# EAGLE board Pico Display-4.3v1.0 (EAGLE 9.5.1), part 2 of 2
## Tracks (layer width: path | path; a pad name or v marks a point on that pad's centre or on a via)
+1V1  (via drill 0.35)
  Top 0.203: U1.50 37.86,33.68 37.86,32.15 39.06,30.94 v39.06,30.61 39.05,30.59 C13.1 | C16.1 33.43,44.09 34.8,44.09 37.06,41.83 37.06,41.3 37.06,41.05 U1.23
  Top 0.254: 37.06,41.3 37.06,40.3 36.59,39.84 36.41,39.84 35.13,38.56 35.13,35.29 35.86,34.56 U1.45 35.86,30.91 v35.52,30.58 35.28,30.34 C14.1
  Bottom 0.5: v39.06,30.61 38.56,30.11 36.25,30.11 35.78,30.58 v35.52,30.58
+3V3  (via drill 0.35, 0.5)  (11 unrouted)
  Top 0.2: U4.8 66.8,57.4 | 69.74,57.4 R53.1 | 28.95,41.17 v29.02,41.17 | v30.91,37.97 31.31,38.37 U1.33 | U3.P$36 64.49,33.41 64.49,33.03 | R46.2 83.7,11.81 R16.2 | U1.44 U1.43 | v64.57,29.55 64.6,29.52 66.96,29.52 C48.1 | R35.2 113.19,25.81 v112.27,25.81
  Top 0.203: U1.10 43.31,38.37 43.55,38.14 v43.69,38.14 v43.69,38.15 44.54,38.15 C10.1 | U1.49 U1.48 37.08,33.91 37.08,31.71 37.49,31.3 | 37.34,29.93 C11.1 37.54,29.73 v37.54,31.27 | C39.1 56.33,37.18 U3.P$12 | C8.1 34.24,44.65 34.77,44.65 37.46,41.97 U1.22 | U1.44 35.3,33.94 | C3.1 43.29,32.95 41.47,34.77 U1.1 | U1.43 35.06,34.44 34.73,34.77 U1.42 | R22.2 44.35,49.9 R21.2 | 64.49,33.03 64.49,31.75 v64.56,31.68
  Top 0.254: U3.P$57 66.59,41.58 68.48,43.47 | 50.24,8.94 C7.1 | 52.8,19.74 53.09,19.46 | R116.2 46.28,54.79 C24.2
  Top 0.3: C18.2 111.25,52.81 111.25,54.38 | 111.25,54.38 111.25,54.76 v110.24,54.76 | 98.73,60.78 101.67,57.83 R118.2 101.78,54.76 v104.14,54.76 | C40.1 68.48,43.78 68.48,43.47 | U13.P$5 111.51,54.64 111.25,54.38 | J10.5 20.91,41.07 | C8.1 34.24,45.16 34.77,45.16 v35.07,45.46 | v45.47,49.94 44.39,49.94 R22.2 | R16.2 84.26,11.76 85.34,12.85 85.34,14.12 84.33,15.14 76,15.14 74.83,16.31 74.83,19.43 74.31,19.95 C37.2
  Top 0.5: C12.1 v33.85,30.89 33.85,32.08 35.26,33.49 35.26,34.16 | J1.3 15.64,63.54 17.27,65.18 18.29,65.18 | 18.29,65.18 18.8,65.18 20.57,63.4 20.57,61.37 21.34,60.6 24.38,60.6 25.53,59.45 C36.1 C47.1 25.53,56.46 26.13,55.86 27.89,55.86 29.1,54.66 C5.1 | R3.2 49.43,55.97 R26.2 49.47,55.49 48.2,54.22 | v44.73,54.15 44.59,54.01 33.97,54.01 v33.76,54.23 31.71,54.23 31.26,54.68 C57.2 29.86,54.67 C5.1 | 31.35,56.96 R74.2 31.35,58.93 32.01,59.59 J2.3 | v71.12,58.06 70.46,57.4 69.74,57.4 66.8,57.4 66.7,57.3 64.77,57.3 63.45,58.62 55.42,58.62 54.31,57.51 R9.2 R19.2 54.31,55.49 53.46,54.64 53.46,54.63 52.3,53.47 50.05,53.47 49.11,54.42 C58.2 48.01,54.43 C24.2 46.6,54.4 44.97,54.4 v44.73,54.15 | 20.91,41.07 22.19,42.35 U10.8 23.38,43.79 C92.1 | C92.1 R1.2 25.18,45.62 13.46,45.62 12.19,44.35 U10.3 12.19,38.54 C90.2 11.39,36.15 C91.1 11.4,36.04 11.4,33.43 | 9.81,27.58 J5.3 15.75,27.62 C26.2 16.17,27.56 14.93,28.8 14.28,28.8 11.4,31.68 11.4,33.43 | R30.2 C38.1 52.46,34.66 C39.1 55.2,33.27 55.2,28.72 56.1,27.82 R36.2 56.12,25.75 56.49,25.38 R7.2 57.37,25.36 58.05,24.68 v58.05,23.8 | 98.73,60.78 98.73,64.24 97.79,65.18 94.49,65.18 93.4,64.08 J7.14 93.4,58.65 v93.47,58.57 v93.48,58.58 | U2.8 39.55,23.85 39.31,24.09 C15.1 C9.1 | C9.1 | v44.45,31.3 44.15,31.6 C3.1 | R27.2 50.24,8.94 | C7.1 50.64,8.88 53.09,11.33 53.09,19.46 | v39.22,26.64 39.31,26.55 C9.1 | C92.1 25.53,43.64 27.14,42.03 27.12,42 C27.1 27.3,41.17 v29.02,41.17 | C5.1 31.35,54.66 R73.2 31.35,55.86 | v69.44,54.57 69.72,54.29 69.72,45.89 68.6,44.77 C40.1 | 18.29,65.18 v18.29,65.68 | 11.4,33.43 11.14,33.17 v10.41,33.17
  Top 0.5: v44.73,54.15 44.8,54.22 | 49.43,57.72 48.51,58.64 48.51,61.94 J6.3 | v110.49,35.97 R85.2
  Top 0.8: C37.2 C41.2 C44.1 R57.1 R56.1 66.47,19.95 | 66.47,19.95 R59.1 66.42,19.95 | R60.1 62.53,19.77 | R60.1 R58.1 | SD2.4 65.95,16.97 65.2,17.72 65.2,19.95 | 67.1,29.45 C48.1 C49.1 67.07,27.15 66.45,26.54 66.45,26.31 66.47,26.29 R17.2 65.68,26.41 64.82,25.55 64.82,23.52 | C26.2 26.42,27.56 | 26.42,27.56 29.18,27.56 31.23,29.6 C12.1 | R74.2 R73.2 | 52.8,19.74 v58,19.74 36.8,19.74 34.04,22.5 28.45,22.5 26.42,24.54 26.42,27.56 | 59.09,23.75 58.15,23.75 | 64.82,23.52 74.16,23.52 R79.1 76.68,23.64 Q8.2 77.55,23.28 80.68,23.28 R87.1 82.4,24.13 84.07,25.81 87.12,25.81 87.78,25.15 R81.1 C88.1 C35.1 C34.1 93.71,24.57 C33.2 97.9,24.45 L1.2 98.15,22.72 v98.12,22.7 | 64.82,23.52 59.32,23.52 | 61.29,19.96 R58.1 | 61.1,19.74 R58.1 | R60.1 65.2,19.95 | 65.2,19.95 66.47,19.95 | R58.1 61.13,19.77 v58.91,19.77
  Top 1: 59.32,23.52 59.09,23.75
  Bottom 0.2: v30.91,37.97 28.98,39.89 28.98,41.13 v29.02,41.17 | v110.49,35.97 109.97,35.44
  Bottom 0.203: v37.54,31.27 37.49,31.21 35.26,31.21 | v64.56,31.68 64.53,31.65 64.53,29.59 v64.57,29.55
  Bottom 0.254: 109.09,25.76 109.13,25.81 v112.27,25.81
  Bottom 0.3: 45.47,49.68 v45.47,49.94 44.86,49.33 44.86,39.32 v43.69,38.14 | v104.14,54.76 v110.24,54.76
  Bottom 0.5: v93.47,58.57 92.46,59.59 72.64,59.59 v71.12,58.06 69.43,56.37 69.43,54.58 v69.44,54.57 | v33.76,54.23 34.02,53.97 34.02,46.46 35.02,45.46 v35.07,45.46 29.99,45.46 28.68,44.14 28.68,41.52 v29.02,41.17 | v44.73,54.15 44.73,51.18 45.47,50.45 v45.47,49.94 | v44.45,31.3 44.35,31.39 37.67,31.39 v37.54,31.27 37.41,31.39 34.36,31.39 v33.85,30.89 33.85,30.05 36.32,27.58 38.28,27.58 v39.22,26.64 | v10.41,33.17 9.65,32.41 PAD1.P$1 | v110.49,35.97 109.09,34.57 109.09,25.76 109.09,24.5 105.3,20.71 100.12,20.71 v98.12,22.7 | v18.29,65.68 PAD19.P$1
  Bottom 0.8: P13.P$1 57.89,23.64 v58.05,23.8
  other vias: 58.92,18.72 58.01,18.72 58.92,23.77 58.97,22.64 58.04,22.66
  pour Top: 57.71,24.09 57.71,22.56 57.9,22.37 59.16,22.37 59.31,22.51 59.31,24.14 59.03,24.42 58.04,24.42
  pour Bottom (no thermals): 57.46,23.84 57.46,18.77 57.87,18.37 59.12,18.37 59.49,18.74 59.49,23.96 59.03,24.42 58.04,24.42
  pour Top: 57.45,19.96 57.45,18.79 57.88,18.35 58.89,18.35 59.25,18.71 59.25,20.01 59.1,20.16 57.65,20.16
  pour Top: 24.64,27.84 28.19,27.84 28.45,27.58 26.67,25.81 26.16,25.81 24.64,27.33
  pour Top (no thermals): 16.51,27.33 12.95,27.33 12.7,27.58 14.05,28.93 15.41,28.93 16.51,27.84
  pour Top: 51.93,19.68 54.33,19.68 53.13,18.48
+5V  (via drill 0.35)  (7 unrouted)
  Top 0.5: D8.A 109.63,20.19
  Top 0.55: 113.82,18.96 114.63,18.96 115.82,17.77 115.82,15.35 114.65,14.17 113.56,14.17
  Top 0.6: 113.51,18.97 112.24,18.97 112.14,19.08 | 113.56,14.12 v112.27,14.12
  Top 0.8: 112.14,19.08 111.38,19.08
  Top 1: 111.38,19.08 110.19,20.26 D8.A 109.55,20.34 109.55,22.89
  Bottom 0.5: PAD28.P$1 112.27,15.65 v112.27,14.12
BAT+  (via drill 0.35)  (1 unrouted)
  Top 0.2: 97.79,38.29 v97.81,38.31
  Top 0.5: 108.78,30.89 109.22,30.89 | C19.2 101,37.39 Q19.3 97.79,38.29
  Top 0.8: 108.78,30.89 106.44,33.23 106.44,34.65 105.46,35.63 U26.3 105.28,36.52 C20.2 C19.2
  Top 1: D14.A 110.09,31.87 J16.P$1
  Bottom 0.2: PAD53.P$1 99.28,38.31
  Bottom 0.5: v97.81,38.31 99.28,38.31
BL-POWER  (via drill 0.35)
  Top 0.2: U3.P$25 60.06,32.22 v58.37,30.53 | R50.2 95.48,44.76 95.48,32.47 97.75,30.2 97.75,27.12 96.32,25.68 v95.48,25.68 | v93.66,17.12 v77.35,17.12
  Bottom 0.2: 95.48,25.61 v95.48,25.68 95.48,24.93 94.02,23.47 94.02,17.47 v93.66,17.12 | v58.37,30.53 58.37,30.13 57.2,28.96 53.12,28.96 51.19,27.02 51.19,17.5 51.75,16.94 58.66,16.94 62.08,20.36 71.94,20.36 75.11,17.19 77.28,17.19 v77.35,17.12
BL-PWM1
  Top 1: R101.2 R8.1 R4.1 R118.1
BOOT  (via drill 0.35)
  Top 0.2: R6.2 54.92,25.61 54.36,25.61 53.86,25.11 v53.86,24.83 | 107.66,2.09 116.8,11.22 116.8,22.51 118.44,24.15 118.44,25.8 116.44,27.79 116.44,48.2
  Top 0.203: v55.37,18.44 55.37,10.96 58.38,7.95 75.38,7.95 81.24,2.09 107.66,2.09
  Top 0.254: 116.44,48.2 115.33,49.32 SW2.2
  Bottom 0.203: v55.37,18.44 53.86,19.96 v53.86,24.83
BW16-RX
  Top 0.203: R109.2 23.5,53.1 13.01,53.1 9.69,56.42 9.69,57.9 U10.15
BW16-TX
  Top 0.203: U10.16 8.45,58.15 8.45,56.68 12.77,52.36 22.31,52.36 24.97,49.69 R108.2
CHG_LED
  Top 0.2: U26.1 107.46,37.17 D15.-
D+
  Top 0.203: R11.1 110.39,16.38 111.99,16.38 112.01,16.38 | J14.B6 112.78,17.32 112.42,17.32 112.01,16.92 112.01,16.38 | J14.A6 113.6,16.38 112.01,16.38
D-
  Top 0.203: R10.1 110.32,15.82 J14.B7 114.72,15.82 115.06,16.15 115.06,16.66 114.91,16.82 J14.A7
DVI5V
  Top 0.254: U3.P$9 54.54,38.38 C30.1
  Top 0.8: C30.1 R30.1 R31.1
DVI-CABLE-D  (via drill 0.35)
  Top 0.2: 58.06,31.27 56.87,31.27 56.75,31.39 v56.64,31.39 | R41.1 53.89,30.74 v54.05,30.58
  Top 0.203: U3.P$22 58.84,33.41 58.84,32.05 58.06,31.27
  Bottom 0.2: v54.05,30.58 54.86,31.39 v56.64,31.39
DVI-CABLE-DET
  Top 0.2: R40.1
  Top 0.5: R41.2 R40.1
DVI-CEC  (via drill 0.35)
  Top 0.2: 22.1,33.17 28.9,39.97 U1.29
  Top 0.203: v60.69,30.53 62.06,31.9 U3.P$30 | v52.03,17.73 40.22,17.73 v40.19,17.77 | 22.1,33.17 19.56,33.17 v18.8,33.93
  Bottom 0.203: v52.03,17.73 52.03,27.32 53.31,28.6 58.77,28.6 v60.69,30.53 | v18.8,33.93 18.8,31.14 24.89,25.04 32.91,25.04 v40.19,17.77
DVI-CLKN
  Top 0.2: U1.11 U3.P$8
DVI-CLKP
  Top 0.2: U3.P$7 U1.12
DVI-D0N  (via drill 0.35)
  Top 0.2: U1.13 43.59,39.57 44.4,40.39 44.4,41.02 43.97,41.45 42.92,41.45 v42.67,41.7 | v42.46,46.88 42.54,46.88 42.78,46.64 52.78,46.64 55.12,44.3 55.12,43.28 56.82,41.58 U3.P$1
  Bottom 0.2: v42.67,41.7 42.42,41.45 41.99,41.45 41.63,41.81 41.63,42.29 43.94,44.6 43.94,46.1 43.41,46.63 42.72,46.63 v42.46,46.88
DVI-D0P  (via drill 0.35)
  Top 0.2: U3.P$2 56.52,41.18 54.77,42.93 54.77,44.11 52.63,46.25 42.82,46.25 42.82,46.23 v42.57,45.98 | v42.67,40.79 42.67,40.89 42.82,41.05 43.69,41.05 43.97,40.77 43.97,40.49 43.43,39.95 41.11,39.95 U1.14
  Bottom 0.2: v42.57,45.98 42.57,46.03 42.77,46.23 43.23,46.23 43.51,45.95 43.51,44.68 41.28,42.45 41.28,41.58 41.81,41.05 42.42,41.05 v42.67,40.79
DVI-D1N  (via drill 0.35)
  Top 0.2: U3.P$3 56.09,40.78 53.78,43.09 47.35,43.09 v47.09,43.34 | U1.15 40.26,41.18 41.87,42.79 44.23,42.79 44.96,42.06 44.96,41.78 46.23,40.51 46.84,40.51 v47.17,40.18
  Bottom 0.2: v47.17,40.18 46.83,40.51 46.23,40.51 45.7,41.05 45.7,42.7 46.1,43.1 46.85,43.1 v47.09,43.34
DVI-D1P  (via drill 0.35)
  Top 0.2: U3.P$4 55.98,40.38 53.67,42.69 47.37,42.69 v47.09,42.41 | U1.16 39.86,41.28 41.76,43.18 44.6,43.18 45.44,42.34 45.44,41.82 46.37,40.89 46.91,40.89 v47.13,41.11
  Bottom 0.2: v47.13,41.11 46.89,40.87 46.41,40.87 46.05,41.23 46.05,42.44 46.3,42.7 46.85,42.7 47.09,42.45 v47.09,42.41
DVI-D2N  (via drill 0.35)
  Top 0.2: U1.17 39.5,40.86 39.5,41.62 42.48,44.59 51.86,44.59 v52.18,44.27 | U3.P$5 53.06,39.98 52.55,40.49 52.55,40.79 52.8,41.05 52.97,41.05 53.32,40.69 v53.32,40.66
  Bottom 0.2: v52.18,44.27 52.44,44.52 52.67,44.52 52.95,44.24 52.95,43.5 51.9,42.45 51.9,41.71 52.57,41.04 52.94,41.04 v53.32,40.66
DVI-D2P  (via drill 0.35)
  Top 0.2: U1.18 39.06,41.75 42.28,44.97 51.98,44.97 v52.19,45.18 | U3.P$6 52.95,39.58 52.15,40.39 52.15,40.99 52.56,41.4 53.14,41.4 v53.35,41.61
  Bottom 0.2: v52.19,45.18 52.46,44.91 52.87,44.91 53.46,44.31 53.46,43.37 52.36,42.27 52.36,41.83 52.77,41.43 53.17,41.43 v53.35,41.61
DVI-HPD  (via drill 0.35)
  Top 0.203: U1.35 32.19,37.57 30.37,35.76 28.34,35.76 23.85,31.27 v21.34,31.27 | v78.23,7.01 78.23,10.53 Q2.3 80.52,10.56 R43.1 C51.1
  Bottom 0.2: v21.34,31.27 26.67,25.94 33.53,25.94
  Bottom 0.203: 33.53,25.94 52.45,7.01 v78.23,7.01
DVI-HPD0  (via drill 0.35)
  Top 0.2: v82.08,14.2 82.19,14.09 R44.2 | U3.P$63 63.26,43.36 64.15,44.25 65.04,44.25 67.31,46.52 v67.31,47.84
  Top 0.254: R44.2 83.67,13.21 R16.1 | v86.48,14.04 86.52,14 v96.46,14
  Bottom 0.254: v67.31,47.84 67.4,47.74 78.47,47.74 78.96,48.23 96.08,48.23 102.36,41.95 102.36,36.74 99.36,33.74 99.36,25.55 95.9,22.09 95.9,14.56 v96.46,14 | v82.08,14.2 86.32,14.2 v86.48,14.04
EN-TP  (via drill 0.35)
  Top 0.2: U3.P$60 64.46,42.95 64.62,43.1 | 29.5,48.7 28.92,48.12 27.09,48.12 R18.2 | 65.99,43.1 66.66,43.1 67.21,43.66 67.21,44.82 68.61,46.22 | 29.5,50.89 30.2,51.59 32.84,51.59 33.68,52.43 42.46,52.43 43.17,51.72 53.6,51.72
  Top 0.203: 64.62,43.1 65.99,43.1 | 29.5,48.7 29.5,50.89 | v63.47,53.02 54.9,53.02 53.6,51.72 | v68.37,52.84 68.61,52.6 68.61,46.22
  Bottom 0.203: v63.47,53.02 68.19,53.02 v68.37,52.84
EN_RESET  (via drill 0.35)
  Top 0.2: U3.P$61 64.06,43.13 64.4,43.47 | v67.92,48.61 67.96,48.57 67.96,46.23 66.79,45.05 66.79,43.75 66.51,43.47 | R88.2 75.18,35.93 78.08,38.82 78.08,48.29 v78.22,48.43
  Top 0.203: 66.51,43.47 64.4,43.47
  Bottom 0.2: v78.22,48.43 68.1,48.43 v67.92,48.61
FLASH-WP  (via drill 0.35)
  Top 0.2: U3.P$58 66.68,42.53 67.56,43.42 67.56,44.53 69.19,46.16
  Top 0.203: v68.35,55.02 68.35,53.97 69.19,53.13 69.19,46.16 | R20.2 R19.1 56.56,54.87 56.61,54.86 U4.3 58.78,55.11 61.94,55.11 v62.08,54.97
  Bottom 0.203: v68.35,55.02 68.3,55.07 62.17,55.07 v62.08,54.97
GND  (via drill 0.35)  (492 unrouted)
  Top 0.203: C28.2 53.66,49.49 v53.59,49.43 | X1.2 39.91,48.99 40.69,48.2 40.69,44.66 38.66,42.62 U1.19 38.66,38.37 U1.EPAD | C16.2 C8.2 34.59,46.43 v35.13,46.96 | v38.1,44.09 38.02,44.17 C1.2 38.02,46.75 X1.4 39.69,48.49 X1.2 | X1.2 39.97,49.28 v41.45,49.28 42.43,49.28 R23.2 43.12,49.85 43.82,49.15 45.65,49.15 C6.2 47.29,49.2 48.28,49.2 48.98,49.9 C25.2 C21.2 51.85,49.9 v52.32,49.43 | C47.2 C36.2 27.06,59.71 v26.67,60.1 | C57.1 C5.2 | R15.1 27.33,53.57 v28.06,54.3 | C4.2 28.16,45.62 v28.96,45.62 | C92.2 28.53,42.32 v30.59,42.32 | v26.8,39.85 26.74,39.85 C27.2 23.36,38.76 v22.1,38.76
  other vias: 60.35,45.8 63.47,47.9 62.55,50.81 53.74,52.98 55.44,50.87 54.1,48.16 55.98,46.79 58.17,45.62 60.68,51.13 58.93,37.85 58.93,40.74 38.1,65.68 24.89,23.01 31.5,20.98 9.65,50.95 14.48,17.93 35.81,51.21 9.55,48.46 36.93,43.41 59.44,46.71 35.1,48.69 21.89,50.04 45.52,18.8 35.16,61.57 56.96,43.15 14.27,18.9 40.18,50.55 41.25,47.27 38.05,51.41 52.02,12.8 69.25,42.86 70.1,41.07 71.88,40.31 73.66,39.55 75.07,38.62 39.88,43.82 70.61,16.66 72.14,16.66 73.66,16.66 36.83,16.66 36.58,12.85 36.32,8.53 52.32,5.74 50.8,3.71 42.16,14.38 50.29,5.99 11.94,19.46 9.4,39.27 9.4,34.44 18.8,63.4 35.73,65.36 40.49,62.52 38.74,62.54 9.65,53.75 50.29,59.59 57.86,51.28 56.9,54 95.76,63.91 100.84,60.86 102.26,60.76 100.84,63.14 102.62,63.14 103.63,60.86 113.18,62.53 111.66,66.34 113.44,59.23 103.28,56.69 109.37,50.09 101.5,46.28 97.98,47.68 105.31,42.72 97.69,43.23 105.31,38.4 106.58,38.4 107.53,35.02 106.58,37.39 97.69,35.86 97.55,34.39 113.18,24.69 111.91,21.39 113.18,21.89 111.91,22.91 113.18,23.42 20.78,25.4 18.64,25.4 111.91,24.18 112.93,10.97 110.77,11.32 111.19,13.17 103.3,13.9 99.9,14.6 97.25,14.7 107.95,11.28 85.46,10.21 108.67,7.46 111.03,9.25 105.82,17.32 105.36,13.97 84.86,24.28 92.1,21.89 97.19,21.88 84.99,19.61 87.27,18.59 91.71,15 100.48,10.72 99.21,10.72 83.46,8.69 69.93,28.19 75.19,28.61 73.76,27.18 67.14,31.87 53.37,25.95 55.99,32.12 55.02,37.13 44.7,30.1 45.87,36.88 39.01,22.91 32.41,27.74 31.14,27.74 37.74,26.72 57.66,11.84 50.55,22.25 75.91,13.95 80.52,18.44 44.2,22.76 31.75,31.14 37.36,36.86 38.63,36.86 36.09,38.25 36.09,36.89 58.93,34.95 22.35,56.54 16.76,55.27 11.94,56.29 18.03,50.44 9.65,45.87 49.78,64.67 102.36,59.08 104.67,35.01 113.18,36.37 113.18,35.36 113.18,37.64 113.18,30.53 113.18,29.26 113.18,27.74 75.97,66.34 62.84,54.34 67.65,52.04 89.41,63.65 74.17,65.18 71.37,64.67 69.09,64.67 30.48,59.59 16.26,44.6 100.84,28.85 89.05,3.61 107.09,3.61 110.39,6.15 75.59,3.1 101.5,29.51 37.36,35.53 39.9,35.53 60.33,37.85 60.32,40.74 60.33,34.95 63.12,37.85 63.1,40.74 63.12,34.95 64.52,37.85 64.49,40.74 64.52,34.95 63.1,39.29 64.49,39.29 63.1,36.4 64.49,36.4 60.32,36.4 60.32,39.29 58.93,39.29 58.93,36.4 38.63,35.53 36.09,35.53 61.71,40.74 61.71,39.29 61.72,37.85 61.71,36.4 61.72,34.95 39.9,36.86 39.9,38.19 39.9,39.52 38.63,38.19 37.36,38.19 38.61,39.52 37.36,39.52 63.68,26.25 67.6,36.61 56.53,18.62 57.33,17.75 50.55,18.69 49.28,22.5 54.1,17.68 53.34,7.77 54.36,7.77 53.59,9.55 57.66,13.36 54.1,12.6 85.44,15.09 36.07,3.45 55.63,3.45 66.04,3.45 85.34,4.47 29.74,23.49 31.04,23.44 20.95,44.42 17.65,39.09 20.45,31.72 16.64,31.72 27.18,30.89 25.98,30.61 75.95,11.33 92.86,10.48 100.32,27.36 94.47,35.36 93.01,32.35 84.46,32.5 80.75,32.38 113.28,49.94 108.71,67.72 89.92,68.48 97.79,68.73 82.55,68.73 108.86,61.01 94.23,56.79 94.23,55.27 96.77,56.79 98.55,55.78 97.03,55.52 96.27,53.24 79.25,52.73 82.13,42.75 80.81,40.62 84.36,40.62 87.67,40.62 91.44,40.76 80.84,36.07 84.36,36.08 88.02,36.07 84.7,46.47 98.63,53.42 86.24,43.1 45.97,39.85 54.36,40.63 54.13,43.65 45.8,43.69 52.12,48.01 44.12,43.82 55.69,44.91 35.18,32.26 45.59,24.13 47.97,15.38 63.73,24.7 55.88,64.16 60.45,64.16 93.11,46.82 35.37,39.77 76.53,21.03 83.49,18.97 81.6,19.81 92.59,17.81 46.21,33.21 36.42,54.82 40.79,54.85 46.01,58.63 56.22,22.29 88.87,15.01 52.96,22.67 62.48,24.74 51.4,34.32 56.06,30.43 65.21,28.41 69.03,31.87 67.14,33.52 92.61,8.2 99.79,8.34 105.42,10.62 105.36,8.24 70.79,36.68 77.96,34.58 57.25,30.6 91.52,36.2 62.4,26.33 76.17,35.88 98.67,32.29 89.67,43.09 93,42.99 88.03,32.39 68.02,41.95 70.16,45.17 71.87,46.36 71.87,54.38 67.65,49.87 71.87,49.23 55.64,35.51 55.64,34.11 62.53,31.07 64.46,27.39 62.71,27.78 71.63,42.62 73.1,41.57 74.46,40.41 75.97,39.54 78.24,37.87 62.73,29.28 61.61,46.85 51.81,39.83 56.21,43.96 57.46,32.5 32.46,40.71 30.64,40.82 32.6,32.17 28.72,32.29 67.7,35.11 70.89,33.64 69.11,33.57 70.86,35.14 69.17,36.68 80.77,34 80.74,38.34 84.38,38.34 87.74,38.52 91.52,38.55 84.38,34.28 87.95,34.14 69.21,35.21 83.07,22.98 84.72,22.95 75.83,27.74 72.68,24.52 71.09,28.16 78.83,35.04 69.83,29.28 78.91,22.14
  pour Bottom (rank 2, no thermals): 7.87,69.62 113.79,69.62 113.79,1.93 7.87,1.93
  pour Top (rank 2, no thermals): -0.25,72.03 122.17,72.03 122.17,-0.61 0,-0.61 0,33.68 7.87,33.68 7.87,65.43 -0.25,65.43
GP0/UART0_TX  (via drill 0.35)
  Top 0.2: J7.1 56.24,60.95 56.14,60.85
  Top 0.203: U1.2 41.58,35.17 45.48,31.26 46.61,31.26 48.51,29.36 48.51,28.81 v49.24,28.08 | v51.82,54.25 52.53,54.97 R70.1 53.35,56.25 53.35,58.07 56.14,60.85
  Bottom 0.2: v51.82,54.25 53.99,56.42 PAD44.P$1
  Bottom 0.203: v49.24,28.08 49.9,28.74 49.9,50.68 51.56,52.34 51.56,54 v51.82,54.25
GP1/UART0_RX  (via drill 0.35)
  Top 0.2: 62.92,62.2 J7.2
  Top 0.203: U1.3 41.73,35.57 45.59,31.71 46.77,31.71 49.2,29.29 v49.2,29.03 | v50.8,54.25 51.13,54.59 R83.1 50.67,55.4 50.29,55.78 50.29,58.45 55.09,63.25 61.87,63.25 62.92,62.2
  Bottom 0.2: v50.8,54.25 50.8,54.95 PAD43.P$1
  Bottom 0.203: v50.8,54.25 50.8,52.73 49.51,51.44 49.51,29.34 v49.2,29.03
GP2/I2C1_SDA  (via drill 0.35)  (1 unrouted)
  Top 0.2: v65.3,58.65 v65.29,58.65 65.46,58.81 J7.3 65.46,64.34 | U1.4 41.9,35.97 45.77,32.1 47.02,32.1 50.02,29.11 50.41,29.11 v50.61,28.91 | 65.46,64.34 65.53,64.41 | 65.46,64.34 65.46,64.49 v65.28,64.67 | 46.37,62.09 J6.2 | R121.1 v38.49,55.84 v38.5,55.83 39.13,55.83 Q5.3 | J6.2 46.5,65.66 v46.37,65.79 | J6.2 46.5,59.83 47.91,58.43 R3.1
  Top 0.203: R3.1 48.16,57.65
  Bottom 0.2: v65.28,64.67 62.99,66.95 47.53,66.95 | 47.53,66.95 47.52,66.95 | v38.5,55.83 37.06,55.83 36.47,56.42 36.47,61.95 39.83,65.31 45.88,65.31 v46.37,65.79 | v46.37,65.79 | v46.37,65.79 47.53,66.95 | v50.61,28.91 50.63,28.93 50.34,29.23 50.34,50.62 52.19,52.48 52.19,53.57 59.39,60.76 63.18,60.76 v65.3,58.65
GP2/I2C1_SDA-5V  (via drill 0.35)
  Top 0.2: U3.P$71 60.06,44.2 63.14,47.27 63.74,47.27 64.11,47.64 64.11,50.24 62.36,51.99 55.45,51.99 54.38,50.93 41.58,50.93 v41.54,50.96
  Top 0.254: R45.1 41.92,57.42 41.92,58.14 v41.55,58.51 | R121.2 Q5.2 38.73,58.58 v38.78,58.63
  Bottom 0.2: v41.55,58.51 41.51,58.47 41.51,51 v41.54,50.96
  Bottom 0.254: v41.55,58.51 41.36,58.7 38.85,58.7 v38.78,58.63
GP3/I2C1_SCL  (via drill 0.35)  (1 unrouted)
  Top 0.2: v67.92,64.59 67.92,61.37 | 67.92,61.37 67.92,61.03 J7.4 | 47.14,58.46 44.75,60.85 44.75,61.71 J6.1 44.5,65.46 | U1.5 42.01,36.37 45.86,32.53 47.22,32.53 50.12,29.62 50.8,29.62 v51.55,28.88 | v67.56,58.57 68.07,59.08 68.07,61.21 67.92,61.37 | R122.1 34.69,55.84 35.07,55.45 Q9.3
  Top 0.203: R26.1 47.14,56.74 47.14,58.46 | 44.5,65.46 44.5,65.74 v44.7,65.94
  Bottom 0.2: 51.68,28.75 v51.55,28.88 50.75,29.68 50.75,50.53 52.55,52.33 52.55,53.39 59.5,60.34 62.55,60.34 64.87,58.02 67.03,58.02 67.56,58.55 v67.56,58.57 | v33.98,55.83 35.31,55.83 35.95,56.46 35.95,62.09 39.79,65.94 v44.7,65.94
  Bottom 0.203: v67.92,64.59 64.68,67.83 46.6,67.83 v44.7,65.94 43.73,65.94 PAD13.P$1
  Bottom 0.254: v44.7,65.94 44.81,65.94
GP3/I2C1_SCL-5V  (via drill 0.35)
  Top 0.2: U3.P$70 60.45,42.54 60.45,44.05 63.19,46.79 63.87,46.79 64.53,47.45 64.53,50.94 62.99,52.48 55.12,52.48 53.98,51.34 42.59,51.34 42.3,51.63 v42.25,51.57
  Top 0.254: v42.85,60.68 35.44,60.68 32.83,58.07 R122.2 Q9.2 | R47.1 43.41,58.23 v43.12,58.52
  Bottom 0.2: v42.25,51.57 42.25,58.01 42.76,58.52 v43.12,58.52 43.12,60.48 42.92,60.68 v42.85,60.68
GP4/UART1_TX  (via drill 0.35)
  Top 0.203: U1.6 42.4,36.77 45.23,33.95 45.66,33.95 v45.81,34.1 | v28.2,50.92 27.06,50.92 R109.1 27.17,51.19
  Bottom 0.203: v28.2,50.92 25.4,48.11 25.4,39.78 32.2,32.98 44.26,32.98 45.38,34.1 v45.81,34.1
GP5/UART1_RX  (via drill 0.35)
  Top 0.203: U1.7 42.62,37.17 44.53,35.26 45.11,35.26 v45.36,35 | v28.17,49.55 27.2,49.55 R108.1
  Bottom 0.203: v45.36,35 45.36,34.75 44.04,33.43 43.59,33.43 43.57,33.41 32.27,33.41 26.16,39.52 26.16,47.55 v28.17,49.55
GP6/SPI_CLK/SD_CLK  (via drill 0.35)
  Top 0.2: 70.54,64.41 J7.5
  Top 0.203: U1.8 42.72,37.57 44.45,35.84 47.37,35.84 v47.75,35.46 | SD2.5 64.8,15.29 v64.8,16.66 | 70.54,64.41 69.64,65.3 54.99,65.3 53.09,63.4 v51.82,63.4
  Bottom 0.2: 64.8,16.82 v64.8,16.66 64.72,16.66 PAD4.P$1
  Bottom 0.203: 64.86,16.72 v64.8,16.66 | 64.8,16.82 64.25,17.37 60.84,17.37 59.11,15.64 50.73,15.64 47.75,18.62 v47.75,35.46 47.75,36.34 48.67,37.25 48.67,50.55 47.5,51.71 47.5,54.51 51.82,58.83 v51.82,63.4
GP7/SPI_MOSI/SD_SDI  (via drill 0.35)
  Top 0.2: J7.6 73.08,64.74 72.9,64.92
  Top 0.203: U1.9 42.93,37.97 44.65,36.25 48.69,36.25 v48.72,36.21 | SD2.3 v67.05,16.56 67.05,17.51 66.44,18.12 R59.2 | v52.68,64.69 53.92,65.94 71.88,65.94 72.9,64.92
  Bottom 0.203: v67.05,16.56 67.05,17.17 66.33,17.89 62.48,17.89 | 62.48,17.89 60.75,17.89 58.97,16.11 50.88,16.11 48.51,18.48 48.51,36 v48.72,36.21 49.05,36.54 49.05,51.31 48.06,52.3 48.06,54.36 52.68,58.98 v52.68,64.69 | PAD3.P$1 62.48,17.89
GP16/SPI_MISO/SD_SDO  (via drill 0.35)  (1 unrouted)
  Top 0.2: U1.27 35.46,41.28 35.13,41.61 33.42,41.61 30.93,44.09 30.93,48.87 v31.5,49.43 | 75.55,65.24 75.55,61.02 J7.7
  Top 0.203: SD2.7 v62.65,16.66 62.65,18.37 R60.2 | 75.55,65.24 73.89,66.9 34.75,66.9 v34.04,66.19
  Bottom 0.2: v34.04,66.19 31.94,64.1 31.94,49.88 v31.5,49.43 27.81,45.75 27.81,39.4 33.02,34.19 42.93,34.19 44.86,36.12 46.08,36.12 47.37,34.82 47.37,18.29 50.52,15.14 61.12,15.14 v62.65,16.66
GP17/SD_CS/SPI_CS2  (via drill 0.35)
  Top 0.2: U1.28 35.06,41.09 34.93,41.22 33.24,41.22 30.58,43.88 30.58,49.78 v31.24,50.44 | 78.09,64.92 78.09,61.73 77.98,61.62 77.98,61.13 J7.8
  Top 0.203: SD2.2 68.2,15.28 v68.2,16.56 68.2,17.88 68.22,17.9 67.86,18.25 R56.2 | 78.09,64.92 78.09,65.66 76.36,67.38 34.33,67.38 33.52,66.57 v32.94,66.57
  Bottom 0.2: v32.94,66.57 31.24,64.87 v31.24,50.44 27.43,46.63 27.43,39.01 32.68,33.77 43.01,33.77 45.01,35.77 45.9,35.77 46.96,34.7 46.96,18.01 50.25,14.72 67.66,14.72 68.2,15.26 v68.2,16.56
  Bottom 0.203: v68.2,16.56 69.09,17.45 PAD2.P$1
GP19/BUZZER  (via drill 0.35)  (1 unrouted)
  Top 0.2: 28.71,39.26 28.69,39.26 22.25,32.82
  Top 0.203: v17.53,33.17 17.88,32.82 22.25,32.82 | R28.2 39.85,12.66 39.85,15.37 39.85,15.67 v39.37,16.15 | U1.30 29.01,39.57 28.98,39.53 28.72,39.28 28.71,39.26
  Bottom 0.203: v17.53,33.17 17.53,31.14 24.38,24.28 31.75,24.28 39.37,16.66 v39.37,16.15
GP20/I2C0_SDA  (via drill 0.35)
  Top 0.203: U1.31 29.32,39.17 23.34,33.2 23.07,32.92 v23.07,32.67 | J10.1 18.91,36.87 v20.57,35.2
  Bottom 0.2: v23.07,32.67 24.34,31.39 PAD52.P$1
  Bottom 0.203: v23.07,32.67 23.07,32.71 v20.57,35.2
GP21/I2C0_SCL  (via drill 0.35)
  Top 0.203: U1.32 29.83,38.77 v24.03,32.97 | J10.2 19.41,37.64 v20.07,36.98
  Bottom 0.2: PAD16.P$1 20.57,37.49 v20.07,36.98
  Bottom 0.203: v20.07,36.98 20.07,36.68 23.77,32.97 v24.03,32.97
GP22-PWM  (via drill 0.35)  (2 unrouted)
  Top 0.203: J5.1 14.83,23.62 v14.99,23.77 | U1.34 31.88,37.97 30.09,36.19 28.14,36.19 24.13,32.18 24.13,32.16 23.62,31.65 21.85,31.65 21.14,32.36 16.9,32.36 16.82,32.36 v15.49,33.68 | v81.03,67.01 81.03,61.62 80.77,61.37 80.77,61.01
  Bottom 0.203: v14.99,23.77 14.99,25.3 15.49,25.81 v15.49,33.68 15.49,66.19 18.03,68.73 78.49,68.73 80.21,67.01 v81.03,67.01
GP26*ADC0*I2C1_SDA  (via drill 0.35)
  Top 0.2: 83.32,63.24 83.32,61.03 J7.10 | R74.1 29.75,57.41 29.75,61.7 J2.2 29.97,61.99 29.97,63.78 v29.82,63.93 29.9,63.86 40.66,63.86 v40.95,64.14
  Top 0.203: U1.38 32.74,36.37 30.1,33.73 29.36,33.73 v29.21,33.58 | 83.32,63.24 83.31,63.24 v83.31,63.78
  Bottom 0.2: v29.82,63.93 29.82,62.99 PAD8.P$1
  Bottom 0.203: v29.82,63.93 27.71,63.93 23.77,59.99 23.77,37.34 27.53,33.58 v29.21,33.58 | v40.95,64.14 47.3,64.14 48.92,65.76 60.51,65.76 63.07,63.2 82.73,63.2 v83.31,63.78
GP27*ADC1*I2C1_SCL  (via drill 0.35)
  Top 0.2: 29.52,56.35 R73.1 28.01,57.86 28.01,61.62 | J2.1 28.19,62.14 v28.19,64.92 28.52,64.59 31.06,64.59 31.45,64.21 39.76,64.21 v40.1,64.54 | 86.11,63.35 86.11,61.28 J7.11
  Top 0.203: U1.39 32.9,35.97 29.86,32.93 27.67,32.93 v27.64,32.89 | 28.01,61.62 J2.1 | v28.19,64.92 28.25,64.86 | v86.11,63.91 86.11,63.35 86.11,62.89
  Bottom 0.2: v28.19,64.92 27.93,65.19 PAD9.P$1
  Bottom 0.203: v28.19,64.92 23.29,60.02 23.29,37.18 27.58,32.89 v27.64,32.89 | v40.1,64.54 40.35,64.8 47.21,64.8 48.6,66.19 60.96,66.19 63.5,63.65 81.28,63.65 82.04,64.41 85.6,64.41 v86.11,63.91
  Bottom 0.5: PAD9.P$1
GP28-ADC3  (via drill 0.35)  (3 unrouted)
  Top 0.203: J1.1 11.64,62.85 12.06,63.27 v12.06,64.54 12.06,66.07 13.79,67.79 86.79,67.79 88.14,66.45 88.14,61.72 | 34.18,35.56 33.09,35.56 27.39,29.87 15.31,29.87 v13.02,32.16
  Bottom 0.203: v13.02,32.16 13.08,32.21 13.08,61.75 12.06,62.76 v12.06,64.54
LVDS-POWER  (via drill 0.35)
  Top 0.2: v67.39,25.62 66.65,24.89 R17.1
  Top 0.203: U3.P$59 64.86,41.99 65.5,41.36 65.5,34.13 65.92,33.71 65.92,31.75 v65.95,31.71
  Top 0.3: v67.39,25.62 67.53,25.62 R80.2
  Bottom 0.2: v65.95,31.71 65.95,28.18 67.39,26.74 v67.39,25.62
LVDS-RESET  (via drill 0.35)  (2 unrouted)
  Top 0.3: J3.21 84.81,51.59 79.07,45.84 79.07,37.53 78.01,36.47 | C72.1 72.3,33.02 72.3,32.97
  Top 0.35: v77.96,36.49 76.02,34.55 C72.1 73.71,34.55 R88.1
  Bottom 0.2: v77.96,36.49 77.98,36.47 PAD39.P$1
LVDS_3V3  (via drill 0.5)  (1 unrouted)
  Top 0.2: 77.08,31.28 77.08,31.27 77.47,30.89
  Top 0.3: J3.3 J3.2
  Top 0.5: R96.2 73.87,31.41 | R89.2 74.12,33.17 v74.93,33.17
  Top 0.8: R87.2 80.62,25.66 Q8.3 79.59,25.31 77.08,27.82 77.08,31.27 | 73.87,31.41 R89.2 | 94.08,53.09 94.08,36.83 88.55,31.3 77.47,31.3 77.47,30.89 | R96.2 74.01,31.31 77.08,31.28
  Bottom 0.5: PAD21.P$1 v74.93,33.17
  pour Top: 75.95,31.39 78.42,31.39 77.18,30.16
LVDS_LEDA+  (via drill 0.5)  (1 unrouted)
  Top 0.3: J3.25 J3.24 J3.23
  Top 0.6: U5.5 104.74,45.53 v104.65,45.62 | 107.45,52.98 C53.2 C55.2 107.69,51.14 v107.69,50.08 107.69,48.29 D6.C | v104.9,52.98
  Top 0.8: 107.45,52.98 v104.9,52.98
  Top 1: J3.24 v83.31,51.46
  Bottom 0.6: v104.65,45.62 104.65,47.04 v107.69,50.08
  Bottom 0.8: v104.9,52.98 103.38,51.46 v83.31,51.46
LVDS_LEDK-  (via drill 0.5)  (1 unrouted)
  Top 0.2: 100.76,48.97 R99.2
  Top 0.3: J3.29 J3.28 81.53,52.86 J3.27
  Top 0.8: R98.1 102.28,47.46 100.76,48.97 | R99.2 R48.1
  Top 1: J3.28 81.31,49.97 v81.28,49.94 | R99.2 99.39,48.97 98.63,49.73 v98.63,50.06
  Bottom 1: v98.63,50.06 98.45,49.89 81.33,49.89 v81.28,49.94
N$1
  Top 0.203: X1.3 37.32,48.32 C2.2 R2.1
N$2
  Top 0.203: U1.21 37.86,43.4 36.44,44.82 R2.2
N$3
  Top 0.203: U1.20 38.26,43.23 39.55,44.52 C1.1 39.55,46.65 X1.1
N$5
  Top 0.203: J15.B5 106.64,60.26 R68.1
N$8  (via drill 0.35)
  Top 0.2: J3.20 85.31,51.46 79.67,45.82 79.67,34.37 v78.82,33.51
  Top 0.35: R55.1 71.96,31.39 v71.1,32.25
  Bottom 0.2: 78.89,33.58 v78.82,33.51 78.82,32.85 77.77,31.8 71.55,31.8 v71.1,32.25
N$9
  Top 0.2: R84.1 108.8,33.81 U26.5
N$10
  Top 0.8: U6.3 97.21,20.82 L1.1
N$14
  Top 0.2: U4.7 69.48,56.13 R53.2
N$15
  Top 0.2: D15.+ 110.5,38.69 R85.1
N$16
  Top 0.203: J15.A5 109.64,61 R69.2
N$23  (1 unrouted)
  Top 0.254: Q4.1 40.08,10.87 39.88,11.07 | R29.2 39.62,10.88 R28.1
N$27
  Top 0.2: R32.1 100.07,34.79 | Q19.1 99.99,36.39
  Top 0.5: R66.2 R32.1
  Top 0.8: Q19.1 100.19,36.37 R66.2
N$28
  Top 0.203: R12.1 110.32,18.32 J14.B5
N$29  (1 unrouted)
  Top 0.254: Q4.3 39.19,7.22 40.01,7.22 42.3,7.22 | 42.55,10.15 D2.A
  Top 0.5: D2.A 42.53,7.66 42.93,7.26 42.77,7.26 B1.2
N$30
  Top 0.254: R27.1 48.68,7.22 | 46.56,10.16 D2.C
  Top 0.5: R27.1 46.62,7.41 B1.1 46.55,10.15 46.56,10.16
N$31
  Top 0.2: U5.3 103.82,46.99
  Top 0.8: 103.82,46.99 103.82,48.91 R100.1 104.11,49.23 102.68,49.23 R98.2
N$32
  Top 0.203: R13.2 111.08,14.21 112.19,15.32 J14.A5
N$35
  Top 0.3: R35.1 D3.+
N$36
  Top 0.203: R57.2 69.34,18.38 69.34,15.32 SD2.1
N$43  (via drill 0.35)
  Top 0.3: R82.2 R81.2 C88.2 89.86,22.25 89.92,22.25 v89.83,22.16 | v90.32,19.69 90.34,19.69 U6.5
  Bottom 0.3: v89.83,22.16 90.32,21.66 v90.32,19.69
N$49
  Top 0.2: 104.14,50.74 R100.2
  Top 0.8: R101.1 104.14,50.75
  Top 1: 104.14,50.75 104.14,50.74 | R100.2 C73.1
N$50
  Top 0.3: C17.2 113.28,53.49 113.28,58.06 112.9,58.45 U13.P$8
N$51
  Top 0.2: U3.P$29 61.66,32.58 59.88,30.8 59.88,29.63 R38.1
  Top 0.203: U3.P$29 61.64,33.41 | 61.64,29.73 61.33,29.41 R39.2 R38.1
N$52
  Top 0.203: U3.P$23 59.26,33.41
N$57
  Top 0.203: R58.2 61.31,15.47 SD2.8
N$67
  Top 0.203: U3.P$74 58.84,42.55 58.84,43.7 56.42,46.13 55.12,46.13 53.85,47.4 52.51,48.73 50.81,48.73 C21.1 | 48.05,48.63 R21.1 C21.1 | C21.1 C25.1
N$70
  Top 0.5: U5.1 105.74,46.96 105.99,46.71
  Top 1: D6.A 111.91,47.52 L4.2 107.32,45.38 105.99,46.71
N$71
  Top 0.8: Q1.1 98.94,42.82 100.84,42.82 102.1,44.08 Q3.3
  Top 1: Q1.1 96.77,42.11 R49.2
N$73
  Top 0.2: Q3.1 98.39,46.07 R51.2 98.02,45.78 R50.1
N$76
  Top 0.203: R15.2 25.61,53.57 R5.1
N$101
  Top 0.203: U3.P$26 60.46,31.98 59.24,30.76 59.24,29.7 R37.1 57.19,29.35 57.21,29.37 C50.1 56.14,29.37 R36.1
N$102
  Top 0.2: C29.2 R24.1 60.9,49.43 59.51,49.43 X2.3
N$103
  Top 0.2: U3.P$75 58.46,43.29 56.13,45.62 55.04,45.62 53.31,47.35 45.28,47.35 R22.1
  Top 0.203: R23.1 R22.1
N$105
  Top 0.2: R78.1 103.79,42.19 U5.4
N$121
  Top 0.5: Q11.3 74.82,25.71 R79.2 76.2,25.64 Q8.1
N$122
  Top 0.5: Q11.1 71.11,26.37 R86.2 69.65,26.39 R80.1
QSPI_CS  (via drill 0.35)
  Top 0.203: U1.56 40.26,33.68 41.99,31.95 41.99,29.72 42.6,29.11 44.22,29.11 45.47,27.86 45.47,26.82 46.48,25.81 v49.68,25.81 | v49.78,23.77 49.78,23.85 U2.1 51.84,23.61 54.95,23.61 R6.1 R7.1
  Bottom 0.203: v49.68,25.81 49.68,23.88 v49.78,23.77
QSPI_D0
  Top 0.203: U2.5 43.24,27.41 41.52,27.41 40.83,28.1 40.83,31.24 39.06,33.02 U1.53
QSPI_D1
  Top 0.203: U2.2 46.04,25.12 44.96,26.2 44.96,27.84 44.2,28.6 42.42,28.6 41.59,29.43 41.59,31.54 39.86,33.28 U1.55
QSPI_D2  (via drill 0.35)
  Top 0.203: U1.54 39.46,33.17 41.23,31.4 41.23,28.87 v41.86,28.24 | U2.3 50.83,26.39 50.38,26.85 47.98,26.85 45.62,29.21 v45.52,29.21
  Bottom 0.203: v45.52,29.21 44.55,28.24 v41.86,28.24
QSPI_D3
  Top 0.203: U1.51 38.26,32.54 40.03,30.76 40.03,27.68 42.67,25.04 43.41,25.04 U2.7
QSPI_SCK
  Top 0.203: U1.52 38.66,32.79 40.43,31.01 40.43,27.89 41.93,26.39 U2.6
RESET  (via drill 0.35)
  Top 0.2: 35.86,41.42 35.11,42.16 34.42,42.16 v34.25,42.34 | 107.87,1.51 117.16,10.8 117.16,22.26 118.93,24.04 118.93,26.08 116.83,28.18 116.83,48.31 117.01,48.48 117.01,59.69
  Top 0.203: U1.26 35.86,41.42 | v29.72,43.33 27.79,45.26 R1.1 C4.1 25.42,46.84 19.44,46.84 v19.38,46.9 | SW4.2 117.01,59.69 | 107.87,1.51 81.13,1.51 75.12,7.52 57.66,7.52 v56.39,8.79
  Bottom 0.2: v34.25,42.34 33.26,43.33 v29.72,43.33
  Bottom 0.203: v56.39,8.79 52.19,8.79 34.18,26.8 27.71,26.8 19.38,35.13 v19.38,46.9
RP2040-BL-PWM  (via drill 0.35)
  Top 0.2: U1.36 32.45,37.17 30.18,34.9 v28.63,34.9 | R4.2 101.94,53.75 v103.12,53.75 | v28.16,52.43 28.61,51.98 32.57,51.98 33.62,53.03 42.77,53.03 43.71,52.09 48.91,52.09 v49.19,52.36
  Bottom 0.2: v103.12,53.75 103.12,55.4 97.06,61.46 56.49,61.46 54.48,59.46 53.84,59.46 49.19,54.8 v49.19,52.36 | v28.63,34.9 24.64,38.89 24.64,50.19 26.4,51.95 28.06,51.95 28.16,52.05 v28.16,52.43
RTD3V1  (via drill 0.35)
  Top 0.2: U3.P$68 61.26,44.24 63.31,46.29 | R14.1 99.63,56.92 v97.92,56.92
  Top 0.203: 63.31,46.29 63.95,46.29 64.91,47.25 64.91,52.59 63.85,53.65 61.29,53.65 v60.91,54.04
  Bottom 0.2: v60.91,54.04 60.91,54.84 61.71,55.65 67.61,55.65 72.06,60.1 94.74,60.1 v97.92,56.92
RTD3V3
  Top 0.254: R47.2 R117.1
  Top 0.5: R47.2 43.31,55.82 R45.2 | R116.1 R117.1
RTD2281-BL-PWM  (via drill 0.35)
  Top 0.2: R8.2 101.81,52.22 102.36,52.22 102.95,52.81 v103.05,52.81 | 57.26,31.78 56.5,32.53 v56.5,33.31
  Top 0.203: U3.P$21 58.46,32.29 57.96,31.78 57.26,31.78
  Bottom 0.2: v103.05,52.81 102.36,53.49 102.36,55.58 96.83,61.11 71.25,61.11 67.68,57.54 67.67,57.56 64.76,57.56 62.54,59.78 59.5,59.78 52.93,53.21 52.93,51.68 51.17,49.92 51.17,35.5 53.4,33.27 56.47,33.27 v56.5,33.31
RX  (via drill 0.35)
  Top 0.203: v54.86,62.13 51.18,58.45 51.18,56.98 R83.2
  Top 0.254: U13.P$6 109.6,55.91 v109.47,56.03
  Bottom 0.203: v54.86,62.13 55.12,62.38 106.43,62.38 109.47,59.33 v109.47,56.03
RX-DOWNLOAD
  Top 0.5: U10.5 16.19,41.08 P82.P$1
SCL  (via drill 0.35)
  Top 0.2: v70.63,30.12 70.17,30.58 63.85,30.58 63.26,31.17 U3.P$33
  Bottom 0.254: v70.63,30.12 71.01,30.51 96.17,30.51 97.65,29.03 97.65,26.57 94.39,23.31 94.39,6.6 J4.P$3
SDA  (via drill 0.35)
  Top 0.254: v70.45,31.36 70.45,31.25 70.2,31 64.09,31 63.66,31.43 U3.P$34
  Bottom 0.254: v70.45,31.36 96.65,31.36 98.44,29.57 98.44,26.03 95.13,22.72 95.13,8.4 J4.P$2
SPI-CE
  Top 0.2: U3.P$67 61.66,44.03 63.52,45.88 | 60.59,57.4 62.23,57.4 63.07,56.56 63.07,55.07 65.31,52.83
  Top 0.203: 63.52,45.88 64.19,45.88 65.31,47 65.31,52.83 | 60.74,57.4 60.59,57.4 U4.1 56.16,57.4 R9.1
SPI-CLK
  Top 0.2: U3.P$64 62.86,43.46 | 67.85,54.02 67.85,53.3 66.53,51.98 66.53,46.47
  Top 0.203: 62.86,43.46 64.01,44.61 64.67,44.61 66.53,46.47 | 67.85,54.02 67.01,54.86 U4.6
SPI-SDIN
  Top 0.2: U3.P$65 62.46,43.6 63.83,44.96
  Top 0.203: 63.83,44.96 64.43,44.96 66.14,46.68 66.14,53.1 U4.5
SPI-SDOUT  (via drill 0.35)
  Top 0.2: U3.P$66 62.06,43.85 63.53,45.32
  Top 0.203: 63.53,45.32 64.23,45.32 65.73,46.82 65.73,52.98 63.78,54.93 v63.78,56.42 | v60.79,56.35 58.75,56.35 U4.2
  Bottom 0.203: v63.78,56.42 63.43,56.07 61.07,56.07 v60.79,56.35
SWCLK
  Top 0.203: U1.24 36.66,41.67 34.68,43.65 32.48,43.65 31.78,44.35 31.78,47.19 P11.P$1
SWDIO
  Top 0.203: P12.P$1 31.36,48.26 31.36,44.2 32.33,43.23 34.59,43.23 36.26,41.57 U1.25
TE  (via drill 0.35)
  Top 0.2: U3.P$62 63.66,43.24 64.26,43.84 | v66.05,44.26 65.63,43.84 65.28,43.84 | v94.47,32.59 94.47,32.1 92.86,30.49 78.82,30.49 v78.08,29.76 | v75.46,29.82 73.97,29.82 R96.1
  Top 0.203: 64.26,43.84 65.28,43.84
  Top 0.5: R55.2 72.39,28.51 R97.2 73.26,29.22 R96.1
  Bottom 0.2: PAD38.P$1 66.05,46.09 v66.05,44.26 66.05,46.87 66.33,47.15 78.48,47.15 79,47.68 95.89,47.68 101.75,41.83 101.75,36.85 97.45,32.56 94.51,32.56 v94.47,32.59 | v78.08,29.76 75.53,29.76 v75.46,29.82
TMDS3V1
  Top 0.2: Q2.1 79.67,13.21 R44.1 R46.1
TP-EN  (via drill 0.35)
  Top 0.2: 19.23,41.38 19.3,41.3 19.52,41.08 | v18.54,44.33 18.54,44.35 v18.54,44.33 | v18.54,44.33 18.97,43.9 18.97,41.63 | v18.54,48.07 18.63,48.16 R18.1 | U1.37 34.17,36.73 32.54,36.73 30.08,34.26 28.02,34.26 24.38,30.63 16.26,30.63 14.22,32.66 14.22,37.49 17.71,40.98 19.36,40.98 | 19.36,40.98 19.6,40.98 | 19.52,41.08 19.91,40.7 J10.3 | 19.36,40.98 19.46,41.08 19.52,41.08
  Top 0.203: 19.3,41.3 18.97,41.63
  Bottom 0.2: v18.54,44.33 v18.54,48.07
  Bottom 0.203: v18.54,48.07 19.73,49.26 PAD51.P$1
TP-RESET  (via drill 0.35)
  Top 0.2: J10.6 21.41,37.92 22,37.33 22,36.24 22.66,35.58 v22.86,35.58 | v30.5,31.74 30.5,32.26 33.43,35.19 34.2,35.19 U1.41
  Bottom 0.2: v22.86,35.58 23.11,35.58 27.05,31.65 30.41,31.65 v30.5,31.74
  Bottom 0.203: PAD42.P$1 30.5,31.31 v30.5,31.74
TX  (via drill 0.35)
  Top 0.203: v54.86,60.86 52.58,58.57 52.58,56.9 R70.2
  Top 0.254: U13.P$7 108.58,57.18 v108.46,57.3
  Bottom 0.203: v108.46,57.3 108.46,59.33 105.92,61.87 55.88,61.87 v54.86,60.86
TX-DOWNLOAD  (2 unrouted)
  Top 0.203: R5.2 19.56,55.02 17.96,56.62 17.96,59.15
TXE0+  (via drill 0.35)
  Top 0.2: 74.73,58.42 71.24,54.93 71.24,43.27 68.75,40.78 U3.P$55
  Top 0.203: 74.73,58.42 88.54,58.42 91.81,55.15 J3.7 91.81,46.26 92.46,45.62 92.46,44.6 v92.96,44.09
  Bottom 0.203: PAD24.P$1 94.23,42.82 v92.96,44.09
TXE0-  (via drill 0.35)
  Top 0.2: 75.95,58.8 74.41,58.8 70.87,55.26 70.87,43.43 68.61,41.18 U3.P$56
  Top 0.203: 75.95,58.8 88.92,58.8 92.31,55.41 J3.6 92.31,46.52 92.81,46.02 92.81,45.45 v93.15,45.11
  Bottom 0.2: v93.15,45.11 93.22,45.11 PAD23.P$1
TXE1+  (via drill 0.35)  (1 unrouted)
  Top 0.2: 87.96,57.25 75.49,57.25 72.94,54.7 72.94,42.31 70.61,39.98 U3.P$53
  Top 0.203: 87.96,57.25 90.31,54.9 J3.10 90.31,45.73 90.68,45.36 v90.68,44.86
  Bottom 0.203: 89.96,46.29 89.96,46.09 90.68,45.36 v90.68,44.86
TXE1-  (via drill 0.35)
  Top 0.2: U3.P$54 70.46,40.38 72.57,42.49 72.57,55.04 75.13,57.61
  Top 0.203: 90.81,53.75 90.81,55.01 88.21,57.61 75.13,57.61 | 90.81,53.75 J3.9 | 90.81,53.75 90.81,45.99 91.36,45.44 91.36,44.17 v91.44,44.09
  Bottom 0.203: v91.44,44.09 PAD26.P$1 91.42,42.8
TXE2+  (via drill 0.35)
  Top 0.2: 87.07,56.08 76.53,56.08 74.14,53.7 74.14,41.02 72.3,39.18 U3.P$51
  Top 0.203: 87.07,56.08 88.81,54.34 J3.13 88.81,45.97 87.75,44.9 87.57,44.9 v87.39,45.08
  Bottom 0.2: v87.39,45.08 86.48,45.99 PAD31.P$1
  Bottom 0.203: v87.39,45.08 87.14,45.33
TXE2-  (via drill 0.35)  (1 unrouted)
  Top 0.2: 87.3,56.49 76.32,56.49 73.79,53.96 73.79,41.2 72.17,39.58 U3.P$52
  Top 0.203: 87.3,56.49 89.31,54.47 J3.12 89.31,45.84 87.88,44.41 v87.88,44.09
  Bottom 0.203: v87.88,44.09 87.88,43.29
TXE3+  (via drill 0.35)  (1 unrouted)
  Top 0.2: 85.44,53.95 78.84,53.95 77.04,52.15 77.04,39.01 75.61,37.58 U3.P$47 | J3.19 85.81,49.98 80.69,44.86 v80.52,44.86
  Top 0.203: J3.19 85.81,53.57 85.44,53.95
  Bottom 0.203: v80.52,44.86 79.18,46.2
TXE3-  (via drill 0.35)
  Top 0.2: 85.7,54.31 78.49,54.31 76.63,52.45 76.63,39.23 75.39,37.98 U3.P$48 | J3.18 86.31,49.64 81.28,44.6 v81.28,44.09
  Top 0.203: J3.18 86.31,53.69 85.7,54.31
  Bottom 0.2: v81.28,44.09 PAD36.P$1 80.01,42.72
TXEC+  (via drill 0.35)  (1 unrouted)
  Top 0.2: 86.17,54.97 77.67,54.97 75.62,52.91 75.62,40.08 73.92,38.38 U3.P$49
  Top 0.203: 86.17,54.97 87.31,53.82 J3.16 87.31,48.1 84.33,45.11 v84.07,45.11
  Bottom 0.203: v84.07,45.11 83.73,45.46
TXEC-  (via drill 0.35)
  Top 0.2: 86.41,55.37 77.5,55.37 75.21,53.09 75.21,40.2 73.79,38.78 U3.P$50
  Top 0.203: 86.41,55.37 87.86,53.92 87.86,52.9 J3.15 | J3.15 87.72,52.76 | 87.72,52.76 87.72,47.74 84.58,44.6 v84.58,44.09 | J3.15 87.72,52.76 | J3.15 87.72,52.76
  Bottom 0.203: 84.37,43.88 v84.58,44.09
  Bottom 0.5: v84.58,44.09 84.58,43.08 PAD33.P$1
UART_USB_D+  (via drill 0.35)  (1 unrouted)
  Top 0.203: J15.A6 108.64,64.49 108.46,64.67 107.8,64.67 107.64,64.51 J15.B6 107.7,63.21 107.7,58.71 107.44,58.45 U13.P$1 104.78,58.45 v104.65,58.57
  Bottom 0.203: v104.65,58.57 104.65,59.7
UART_USB_D-  (via drill 0.35)  (1 unrouted)
  Top 0.203: 108.14,61.87 108.14,58.5 106.82,57.18 U13.P$2 104.78,57.18 v104.65,57.05 | 108.14,61.87 108.14,62.13 J15.A7 | 108.14,61.87 108.97,61.87 109.14,62.05 J15.B7
  Bottom 0.203: v104.65,57.05 104.65,55.89
UART_VBUS  (via drill 0.35)  (6 unrouted)
  Top 0.6: 111.06,61.61 110.79,61.89 110.79,63.12 | 105.99,63.42 105.99,64.31 107.11,65.43 109.62,65.43 110.79,64.27 110.79,63.42
  Top 0.8: v112.01,28.09 111.56,28.55 D7.A | v112.01,61.62 v112.01,61.61 111.06,61.61
  Top 1: D7.A 109.53,25.87 D1.A
  Bottom 0.8: v112.01,61.62 112.04,61.6 112.04,28.12 v112.01,28.09
  other vias: 112.01,29.36 112.01,30.38 110.74,61.62 112.78,61.62
  pour Bottom: 112.52,27.33 112.52,30.63 112.27,30.89 111.51,30.89 111.25,30.63 111.25,27.36 111.53,27.08 112.27,27.08
  pour Top: 112.52,27.33 112.52,30.63 112.27,30.89 111.51,30.89 111.25,30.63 111.25,27.36 111.53,27.08 112.27,27.08
  pour Top: 113.03,62.13 110.49,62.13 110.24,61.87 110.24,61.11 110.49,60.86 113,60.86 113.28,61.14 113.28,61.87
  pour Bottom: 113.03,62.13 110.49,62.13 110.24,61.87 110.24,61.11 110.49,60.86 113,60.86 113.28,61.14 113.28,61.87
USB_D+  (via drill 0.35)
  Top 0.203: U1.47 36.66,23.69 38.94,21.41 74.95,21.41 76.12,20.24 76.12,17.05 76.76,16.41 79.95,16.41 80.05,16.41 108.13,16.41 R11.2 107.95,16.76 107.76,16.76 107.69,16.76 v107.39,17.07
  Bottom 0.203: v107.39,17.07 107.19,17.27 PAD45.P$1
USB_D-  (via drill 0.35)
  Top 0.203: U1.46 36.26,23.59 38.91,20.93 74.8,20.93 75.67,20.06 75.67,16.77 76.6,15.84 79.82,15.84 79.87,15.84 108.11,15.84 R10.2 107.53,15.48 v107.19,15.14
  Bottom 0.203: v107.19,15.14 107.19,13.87 PAD46.P$1
VIN  (via drill 0.35)
  Top 0.8: U26.4 103.7,33.81 C22.2 103.38,33.08 v103.38,31.9 100.84,31.9 100.84,32.74 R32.2 100.27,33.31
  Top 1: D1.C 105.5,22.99 D4.C 103.69,22.95 103.38,23.27 v103.38,25.55
  Bottom 1: v103.38,25.55 v103.38,31.9 103.38,32.15
  other vias: 103.38,24.54 103.38,23.52 101.09,31.9 102.11,31.9
  pour Top: 104.14,22.76 104.14,26.06 103.89,26.31 103.12,26.31 102.87,26.06 102.87,22.78 103.15,22.5 103.89,22.5
  pour Bottom: 104.14,22.76 104.14,26.06 103.89,26.31 103.12,26.31 102.87,26.06 102.87,22.78 103.15,22.5 103.89,22.5
  pour Bottom: 103.89,32.66 100.58,32.66 100.33,32.41 100.33,31.65 100.58,31.39 103.86,31.39 104.14,31.67 104.14,32.41
  pour Top (no thermals): 103.12,33.68 101.09,33.68 100.33,32.92 100.33,31.65 100.58,31.39 103.86,31.39 104.14,31.67 104.14,32.66
VIN2
  Top 0.8: U5.6 106.98,43.08
  Top 1: Q1.3 101.57,40.17 C56.2 R78.2 105.82,40.16 C52.2 105.88,40.2 108.91,40.2 L4.1 107.77,43.08 106.98,43.08
VIN+5V  (via drill 0.35, 0.5)
  Top 0.254: R43.2 84.5,10.41 87.17,13.08 100.04,13.08 101.85,11.27 J4.P$1 | R31.2 50.4,36.08 49.07,37.42 47.67,37.42 v47.63,37.38 | R117.2 44.84,57.47 44.84,58.8 v44.91,58.87 44.18,59.6 40.84,59.6 40.26,59.03 | Q9.1 35.96,58.22 37.38,59.64 39.76,59.64 40.26,59.14 40.26,59.03 | 40.51,57.58 Q5.1 40.26,57.61 40.26,59.03
  Top 0.5: v53.65,27.36 53.65,29.1 52.01,30.73 50.39,30.73 49.91,31.22 49.91,32.79 50.25,33.13 R40.2 50.59,33.13 49.77,33.95 49.77,35.46 50.39,36.08 R31.2
  Top 0.8: 103.12,18.18 v102.62,17.68 95,17.68 93.76,18.92 U6.1 92.95,18.92 91.11,20.76 U6.4 90.88,21.05 88.74,21.05 C31.2 88.43,21.04 86.62,21.04 C32.1 78.19,21.02 76.77,22.45 60.67,22.45 v60.65,22.47 | 51.03,36.01 R31.2 | 51.03,33.23 R40.2 | v60.62,26.29 60.33,26.58 60.27,26.58 60.27,27.65 60.13,27.79 | 60.13,27.79 R38.2 | Q1.2 99.95,38.39 Q19.2 | R37.2 60.09,27.83 60.13,27.79
  Top 1: 105.83,20.52 D8.C 103.04,20.26 | Q1.2 96.77,40.11 R49.1 96.27,40.08 96.27,33.01 98.61,30.67 104.84,30.67 D14.C 105.47,28.21 105.83,27.85 105.83,28.2 D7.C 103.44,28.55 101.49,26.6 101.49,21.81 103.04,20.26 | 103.12,18.18 103.04,18.26 103.04,20.26
  Bottom 0.254: v47.63,37.38 48.28,38.03 48.28,50.36 47.01,51.63 47.01,56.63 44.91,58.73 v44.91,58.87
  Bottom 0.5: v102.62,17.68 102.36,17.68
  Bottom 0.8: v53.65,27.36 54.66,26.34 60.62,26.34 v60.62,26.29 60.65,26.25 v60.65,22.47 | 101.85,7.77 101.85,16.92 v102.62,17.68
  Bottom 1: J4.P$1 101.85,7.77
  other vias: 101.35,17.68 100.08,17.68 98.55,17.68 97.28,17.68 60.65,25.11
  pour Top: 97.02,17.17 103.89,17.17 104.14,17.42 104.14,18.19 103.89,18.44 97.08,18.44 96.69,18.06 96.69,17.49
  pour Bottom: 97.05,17.17 103.89,17.17 104.14,17.42 104.14,18.19 103.89,18.44 97.18,18.44 96.69,17.95 96.69,17.53
  pour Bottom: 61.34,24.86 61.34,26.96 61.12,27.19 60.05,27.19 59.86,27 59.86,24.94 60.48,24.32 60.81,24.32
  pour Top: 61.38,24.86 61.38,26.96 61.15,27.19 60.08,27.19 59.9,27 59.9,24.94 60.24,24.6 61.13,24.6
XI
  Top 0.2: C28.1 57.08,47.97 X2.1 59.26,45.78 U3.P$73
XO
  Top 0.2: U3.P$72 59.66,46.02 60.96,47.32 R24.2
(copper drawn outside any net)
  shapes: Top area x2

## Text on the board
tPlace: ADC_GP28 | NC | 3V3 | GND | ADC_GP27 | ADC_GP26 | 3V3 | GND | SCL1_GP3 | SDA1_GP2 | 3V3 | GND | GP | 0 | 1 | 2 | 3 | 6 | 7 | 16 | 17 | 22 | 26 | 27 | 28 | GND | 3V3 | GND | 3V3 | TX0 | RX0 | SDA1 | SCL1 | CLK | MOSI | MISO | CS | PWM | ADC | ADC | ADC | U3 | - | SCL_GP21 | SDA_GP20 | SCL_GP21 | SDA_GP20 | + | GND | 3V3 | NC | PWM-GP22 | V1.0 | GP21-BUZZER | GP6-CLK | GP7-MOSI | GP16-MISO | GP17-CS | GND | SCL | SDA | 5V
tStop: Pico Display-4.3 inch | SKU:DIS01243P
